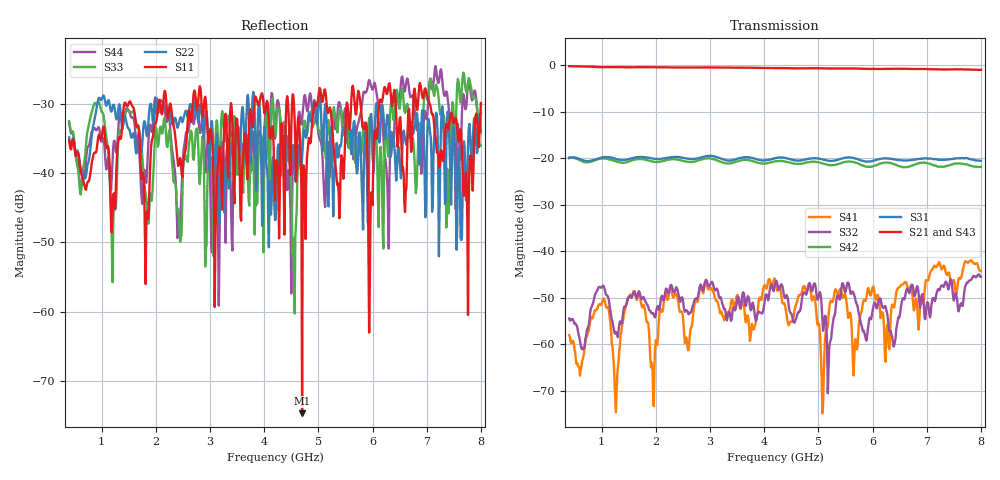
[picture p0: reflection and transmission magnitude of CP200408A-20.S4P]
! Amtery
! Email: info@amtery.com
! Model Number: CP200408A-20
! 4-port S-parameter measurement data for Bi-Directional Coupler
! Frequency Range: 0.4 GHz to 8 GHz
! Port 1: Input
! Port 2: Output
! Port 3: Coupled Forward
! Port 4: Coupled Reverse
# Hz S dB R 50
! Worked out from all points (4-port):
!   609 points, 400 MHz to 8 GHz, reference 50 ohm
!   strongest paths, dB at 400 MHz, 2.3 GHz, 4.2 GHz, 6.1 GHz, 8 GHz:
!     S21: -0.2, -0.4, -0.6, -0.8, -0.9
!     S43: -0.2, -0.4, -0.6, -0.7, -0.9
!     S31: -19.9, -19.7, -19.9, -20.2, -20.5
!     S42: -19.9, -20.2, -20.6, -21.3, -21.8
!     S32: -54.4, -47.7, -46.9, -51.3, -45.5
!     S41: -58.0, -49.1, -46.0, -49.4, -44.3
!   lowest |S11| = -74.6 dB at 4.7 GHz (marker M1), VSWR 1.00, Z = 50 + j0.0075 ohm
!   |S11| at or under -10 dB: start of sweep to end of sweep
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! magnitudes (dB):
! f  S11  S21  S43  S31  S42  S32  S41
! 400 MHz  -35.3  -0.2  -0.2  -19.9  -19.9  -54.4  -58.0
! 4.7 GHz  -74.6  -0.6  -0.6  -20.4  -21.1  -50.1  -48.4
! 5.075 GHz  -29.8  -0.6  -0.6  -20.2  -21.1  -54.5  -74.8
! 5.963 GHz  -46.3  -0.8  -0.7  -20.7  -21.8  -54.6  -49.5
! 6.725 GHz  -36.3  -0.8  -0.7  -20.3  -21.6  -47.1  -48.3
! 7.013 GHz  -29.0  -0.8  -0.8  -20.0  -21.0  -50.9  -46.3
! 8 GHz  -29.9  -0.9  -0.9  -20.5  -21.8  -45.5  -44.3
